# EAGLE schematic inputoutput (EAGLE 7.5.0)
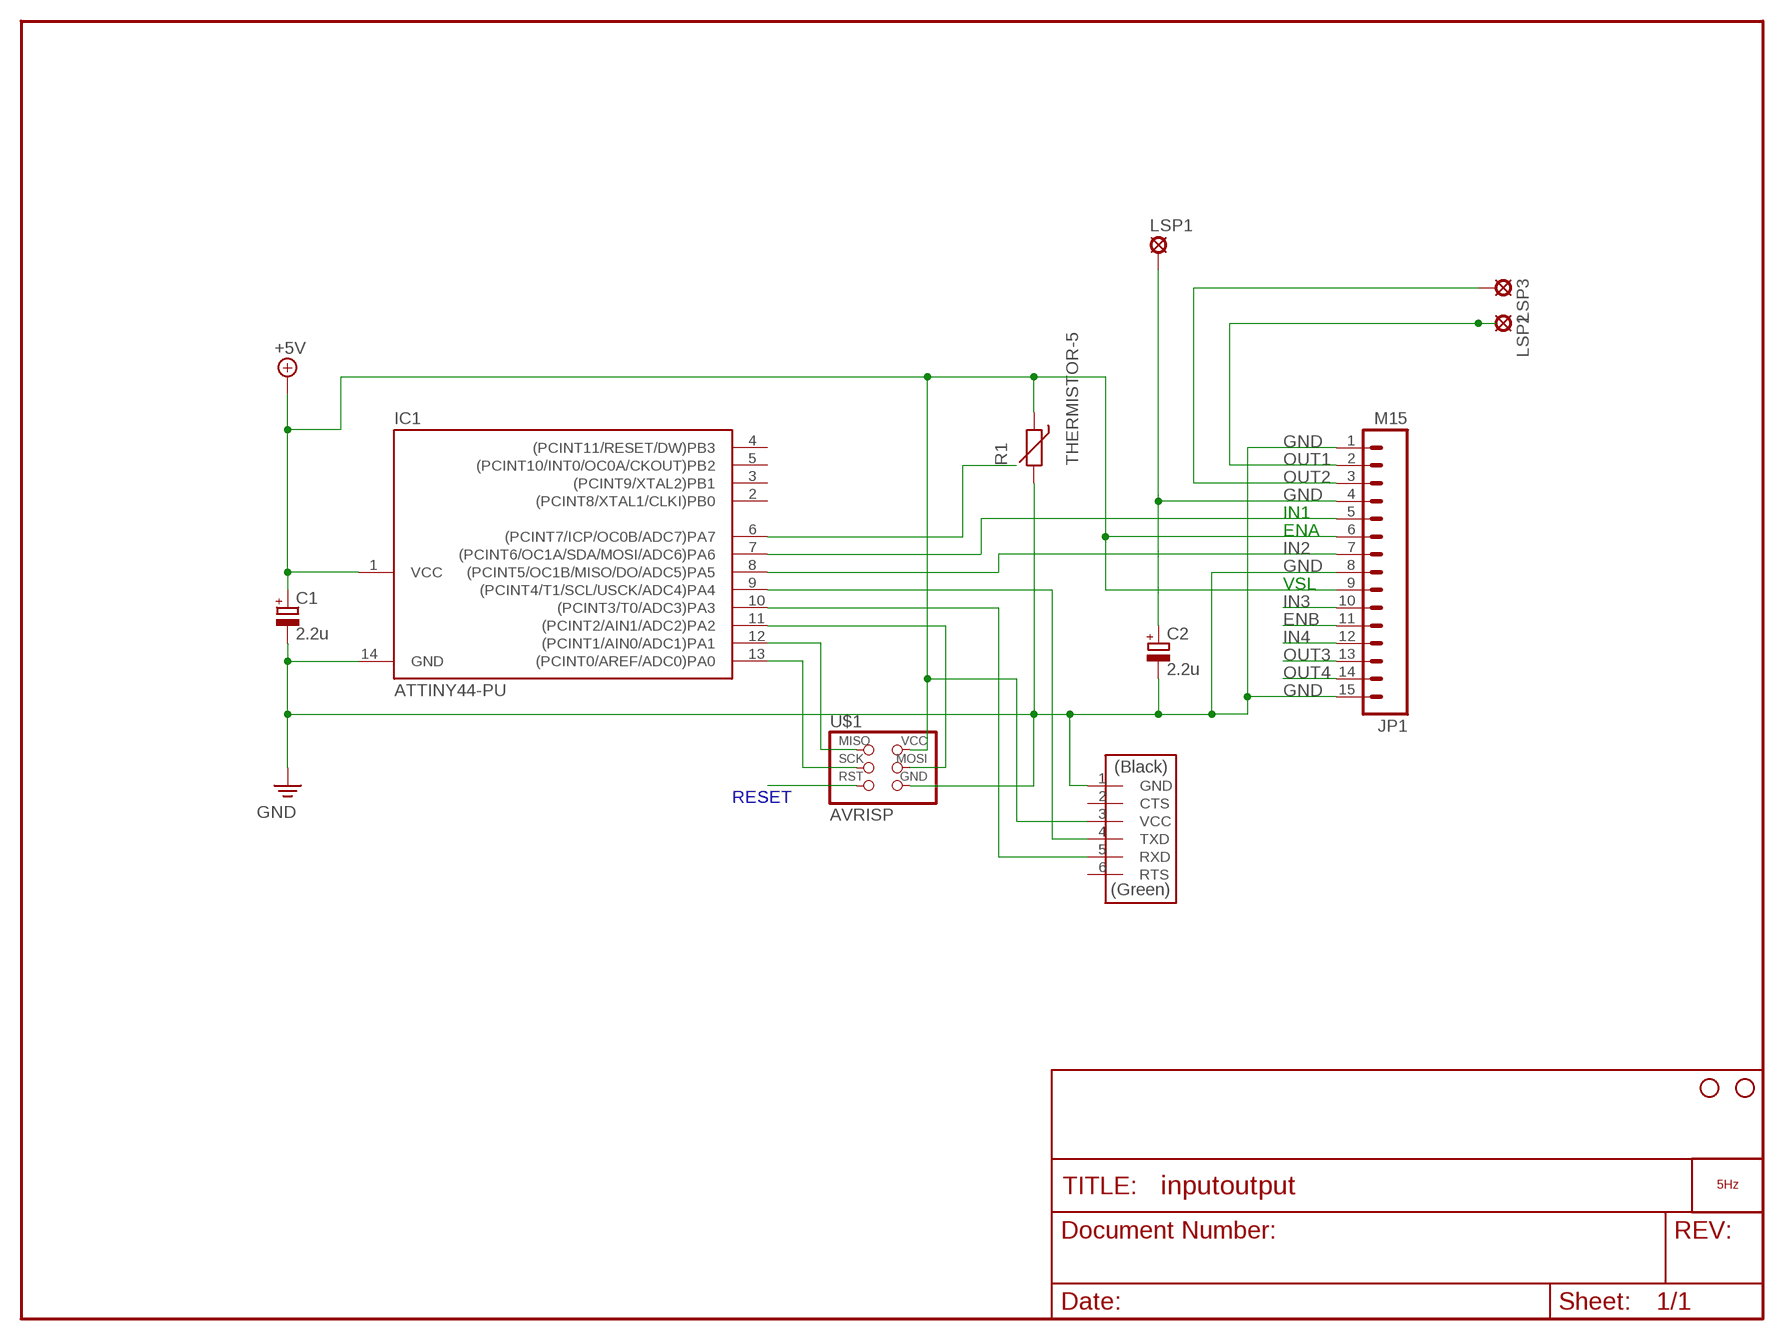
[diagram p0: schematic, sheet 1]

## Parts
C1  2.2u  CPOL-EUC/6032-28R  [C/6032-28R]
C2  2.2u  CPOL-EUC/6032-28R  [C/6032-28R]
IC1  ATTINY44-PU  [DIL14]
JP1  M15  [1X15]
JP2  STAND-OFF  [STAND-OFF]
JP3  STAND-OFF  [STAND-OFF]
LOGO1  LOGO_5HZ_H_20MM  [5HZ_LOGO_H_20MM]
LSP1  LSP13  [LSP13]
LSP2  LSP13  [LSP13]
LSP3  LSP13  [LSP13]
R1  THERMISTOR-5  [R-5]
U$1  AVRISP  [2X03]
U$2  FTDI-SMD-HEADER  [1X06SMD]

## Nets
+5V: C1.+ IC1.1(VCC) JP1.6 JP1.9 R1.1 U$1.2(VCC) U$2.3(VCC)
ENB: JP1.11
GND: C1.- C2.- IC1.14(GND) JP1.1 JP1.8 JP1.15 R1.2 U$1.6(GND) U$2.1(GND)
IN2: IC1.8((PCINT5/OC1B/MISO/DO/ADC5)PA5) JP1.7
IN3: JP1.10
IN4: JP1.12
N$1: IC1.7((PCINT6/OC1A/SDA/MOSI/ADC6)PA6) JP1.5
N$2: C2.+ JP1.4 LSP1.MP
N$3: IC1.6((PCINT7/ICP/OC0B/ADC7)PA7)
N$4: U$1.5(RST)
N$5: IC1.13((PCINT0/AREF/ADC0)PA0) U$1.3(SCK)
N$6: IC1.12((PCINT1/AIN0/ADC1)PA1) U$1.1(MISO)
N$7: IC1.11((PCINT2/AIN1/ADC2)PA2) U$1.4(MOSI)
N$8: IC1.9((PCINT4/T1/SCL/USCK/ADC4)PA4) U$2.4(TXD)
N$9: IC1.10((PCINT3/T0/ADC3)PA3) U$2.5(RXD)
OUT1: JP1.2 LSP2.MP
OUT2: JP1.3 LSP3.MP
OUT3: JP1.13
OUT4: JP1.14
Unconnected: IC1.2((PCINT8/XTAL1/CLKI)PB0) IC1.3((PCINT9/XTAL2)PB1) IC1.4((PCINT11/RESET/DW)PB3) IC1.5((PCINT10/INT0/OC0A/CKOUT)PB2) U$2.2(CTS) U$2.6(RTS)

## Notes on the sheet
- IN1
- ENA
- VSL
- RESET

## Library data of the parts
C1 C2 = rcl:CPOL-EU: POLARIZED CAPACITOR, European symbol
IC1 = fab:ATTINY44
JP1 = SparkFun:M15: Header 15 Standard 15-pin 0.1" header. Use with straight break away headers (SKU : PRT-00116), right angle break away headers (PRT-00553), swiss pins (PRT-00743), machine pins (PRT-00117), and female headers (PRT-00115).
JP2 JP3 = SparkFun:STAND-OFF: Stand Off
LOGO1 = 5hz-electronica:LOGO_5HZ: Logotipo 5Hz "según Pedro"
LSP1-LSP3 = solpad:LSP13: SOLDER PAD
R1 = varistor:THERMISTOR: THERMISTOR
U$1 = fab:AVRISP
U$2 = fab:FTDI-SMD-HEADER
